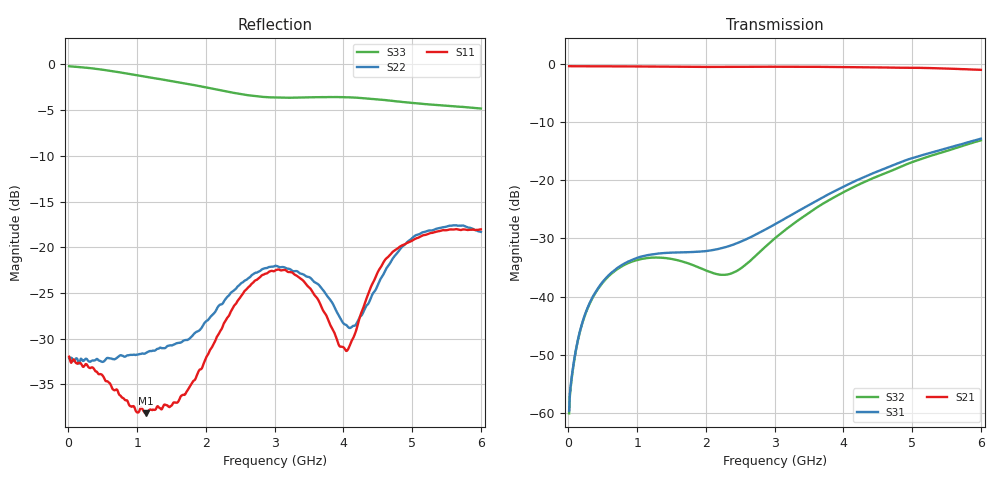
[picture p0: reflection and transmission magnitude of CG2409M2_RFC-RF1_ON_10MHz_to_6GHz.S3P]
!CEL
!CG2409M2
!Port1: RFC Port2: RF1  Port3: RF2
!Freq	S11 S12	S13 S21 S22 S23 S31 S32 S33
# Hz S dB R 50
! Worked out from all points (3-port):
!   600 points, 10 MHz to 6 GHz, reference 50 ohm
!   strongest paths, dB at 10 MHz, 1.51 GHz, 3.01 GHz, 4.51 GHz, 6 GHz:
!     S21: -0.3, -0.4, -0.4, -0.5, -1.0
!     S31: -59.7, -32.4, -27.5, -18.4, -12.8
!     S32: -60.1, -33.5, -29.9, -19.2, -13.1
!   lowest |S11| = -38.2 dB at 1.13 GHz (marker M1), VSWR 1.03, Z = 51.2 - j0.41 ohm
!   |S11| at or under -10 dB: start of sweep to end of sweep
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1e7  -31.97 -5.9  -0.33 -0.3  -59.65 46.3
     -0.33 -0.3  -32.12 -3.4  -60.09 46.4
     -59.66 46.3  -60.11 46.6  -0.18 -1.1
1.4e8  -32.69 -0.7  -0.35 -2.2  -47.33 67.7
       -0.34 -2.2  -32.48 2.7  -47.44 65.6
       -47.31 67.8  -47.45 65.6  -0.27 -10.5
3.5e8  -33.14 0.4  -0.36 -5.1  -40.14 70.8
       -0.35 -5.1  -32.38 -0.1  -40.23 63.5
       -40.13 71.1  -40.26 63.5  -0.43 -25.5
1.13e9  -38.16 -18.9  -0.39 -14.8  -32.92 58.0
        -0.39 -14.8  -31.55 -10.0  -33.40 25.9
        -32.94 58.0  -33.40 25.8  -1.35 -78.3
1.71e9  -35.91 -2.8  -0.44 -21.5  -32.35 60.7
        -0.44 -21.5  -30.14 -0.3  -34.17 -9.4
        -32.36 60.7  -34.17 -9.6  -2.09 -111.0
2.31e9  -27.72 25.9  -0.46 -28.4  -31.41 78.9
        -0.45 -28.4  -25.43 30.4  -36.19 -77.6
        -31.41 78.8  -36.22 -77.5  -2.97 -143.1
3.01e9  -22.53 36.0  -0.43 -36.7  -27.55 98.0
        -0.42 -36.7  -22.03 37.9  -29.95 -156.4
        -27.52 97.9  -29.91 -156.1  -3.62 179.4
4.05e9  -31.33 98.4  -0.47 -50.1  -20.78 100.1
        -0.47 -50.2  -28.56 -29.1  -21.75 157.4
        -20.80 100.0  -21.73 157.4  -3.59 143.5
4.72e9  -20.48 152.3  -0.57 -59.6  -17.41 90.9
        -0.58 -59.7  -21.20 -114.2  -18.19 138.3
        -17.40 90.5  -18.23 138.3  -3.99 125.4
6e9  -18.04 140.5  -0.96 -80.1  -12.96 67.2
     -0.96 -80.3  -18.31 -130.7  -13.19 105.3
     -12.82 67.3  -13.10 105.0  -4.82 88.0
